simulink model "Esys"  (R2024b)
settings: Solver=ode15s  StartTime=0.0  StopTime=0.15  RelTol=1e-6  AbsTol=1e-6  EnableMultiTasking=on
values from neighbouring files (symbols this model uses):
  A = [-1 2; 0 -2]    [cds_matlab_intro_part3.m]    (also in Esys_Parameter.m = [A11,A12;A21,A22]; init_cds_simulink_intro_part1.m = [0 1; -1/T^2 -2*xi/T])
  B = [0;1]    [cds_matlab_intro_part3.m]    (also in init_cds_simulink_intro_part1.m = [0;V/T^2])
  D = 0    [cds_matlab_intro_part3.m]    (also in init_cds_simulink_intro_part1.m)
  te = 0.01    [Esys_Parameter.m]
  ts = 0.03    [Esys_Parameter.m]
  UC1R =     [Esys_Parameter.m]
  UC2R =     [Esys_Parameter.m]
  Ue = 1    [Esys_Parameter.m]
  UeR = 5    [Esys_Parameter.m]
  Us = 4    [Esys_Parameter.m]
  Usinus = 1    [Esys_Parameter.m]
  UsR = 5    [Esys_Parameter.m]
  we = 1e2    (= 100)    [Esys_Parameter.m]

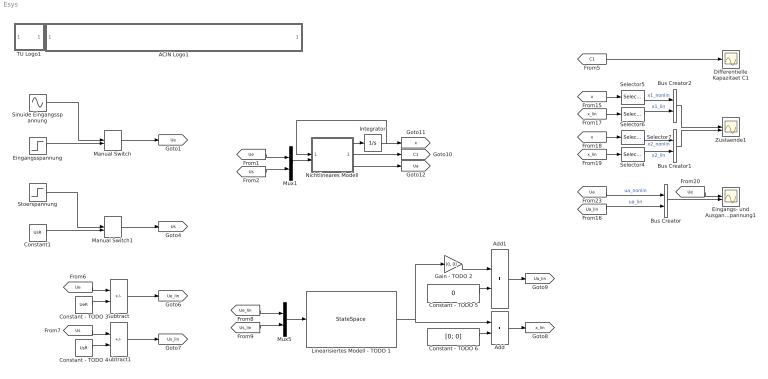
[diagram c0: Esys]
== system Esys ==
  ACIN Logo1 : Subsystem
      mask init:
      | s = get_param(gcb,'UserData');
  Add : Sum
  Add1 : Sum
  Bus Creator : BusCreator  Inputs=2
  Bus Creator1 : BusCreator  Inputs=2
  Bus Creator2 : BusCreator  Inputs=2
  Constant - TODO 3 : Constant  Value=UeR
  Constant - TODO 4 : Constant  Value=UsR
  Constant - TODO 5 : Constant  Value=0
  Constant - TODO 6 : Constant  Value=[0; 0]
  Constant1 : Constant  Value=UsR
  Differentielle Kapazitaet C1 : Scope
  Eingangs- und Ausgangsspannung1 : Scope  NumInputPorts=2
  Eingangsspannung : Step  Time=te  Before=UeR  After=Ue  SampleTime=0
  Gain - TODO 2 : Gain  Gain=[0, 0]  Multiplication=Matrix(K*u)
  Integrator : Integrator  InitialCondition=[UC1R; UC2R]
  Linearisiertes Modell - TODO 1 : StateSpace  A=A  B=B  C=eye(2)  D=[D;D]  InitialCondition=[0;0]
  Manual Switch : ManualSwitch
  Manual Switch1 : ManualSwitch  CurrentSetting=0
  Mux1 : Mux  Inputs=2
  Mux5 : Mux  Inputs=2
  Nichtlineares Modell : MATLAB Function  TreatAsAtomicUnit=on
  Selector4 : Selector  InputPortWidth=2  IndexOptions=Index vector (dialog)  Indices=2  OutputSizes=1
  Selector5 : Selector  InputPortWidth=2  IndexOptions=Index vector (dialog)  Indices=1  OutputSizes=1
  Selector6 : Selector  InputPortWidth=2  IndexOptions=Index vector (dialog)  Indices=1  OutputSizes=1
  Selector7 : Selector  InputPortWidth=2  IndexOptions=Index vector (dialog)  Indices=2  OutputSizes=1
  Sinuide Eingangsspannung : Sin  Amplitude=Usinus  Bias=UeR  Frequency=we  SampleTime=0
  Stoerspannung : Step  Time=ts  Before=UsR  After=Us  SampleTime=0
  Subtract : Sum  Inputs=+-
  Subtract1 : Sum  Inputs=+-
  TU Logo1 : Subsystem
      mask init:
      | s = get_param(gcb,'UserData');
  Zustaende1 : Scope  NumInputPorts=2
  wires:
  Eingangsspannung/1 -> Manual Switch/2
  Sinuide Eingangsspannung/1 -> Manual Switch/1
  Manual Switch/1 -> [Ue]
  [C1] -> Differentielle Kapazitaet C1/1
  Subtract/1 -> [Ue_lin]
  Constant - TODO 3/1 -> Subtract/2
  [Ue] -> Subtract/1
  Subtract1/1 -> [Us_lin]
  Constant - TODO 4/1 -> Subtract1/2
  [Us] -> Subtract1/1
  Linearisiertes Modell - TODO 1/1 -> Gain - TODO 2/1, Add/1
  Mux5/1 -> Linearisiertes Modell - TODO 1/1
  [Ue_lin] -> Mux5/1
  [Us_lin] -> Mux5/2
  Add/1 -> [x_lin]
  Constant - TODO 6/1 -> Add/2
  Gain - TODO 2/1 -> Add1/1
  Constant - TODO 5/1 -> Add1/2
  Add1/1 -> [Ua_lin]
  Manual Switch1/1 -> [Us]
  Stoerspannung/1 -> Manual Switch1/1
  Constant1/1 -> Manual Switch1/2
  Selector7/1 -> Bus Creator1/1  "x2_nonlin"
  Bus Creator/1 -> Eingangs- und Ausgangsspannung1/2
  Bus Creator1/1 -> Zustaende1/2
  Bus Creator2/1 -> Zustaende1/1
  [x_lin] -> Selector4/1
  [x] -> Selector7/1
  Selector6/1 -> Bus Creator2/2  "x1_lin"
  Selector5/1 -> Bus Creator2/1  "x1_nonlin"
  Selector4/1 -> Bus Creator1/2  "x2_lin"
  [Ua_lin] -> Bus Creator/2  "ua_lin"
  [x] -> Selector5/1
  [x_lin] -> Selector6/1
  [Ua] -> Bus Creator/1  "ua_nonlin"
  [Ue] -> Eingangs- und Ausgangsspannung1/1
  [Us] -> Mux1/2
  Mux1/1 -> Nichtlineares Modell/2(u)
  [Ue] -> Mux1/1
  Nichtlineares Modell/1(xp) -> Integrator/1
  Integrator/1 -> Nichtlineares Modell/1(x), [x]
  Nichtlineares Modell/2(C1) -> [C1]
  Nichtlineares Modell/3(Ua) -> [Ua]

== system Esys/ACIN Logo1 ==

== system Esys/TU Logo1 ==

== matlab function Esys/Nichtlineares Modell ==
function [xp, C1, Ua] = fcn(x, u, p)

R1 = p.R1;
R2 = p.R2;
K = p.K;
C1_ref  = p.C1_ref;
C1_inf  = p.C1_inf;
UC1_ref = p.UC1_ref;
C2      = p.C2;

% Shortcut fuer den Eingang
Ue = u(1);
Us = u(2);

% Shortcut fuer die Zustaende
UC1 = x(1);
UC2 = x(2);

% TODO
Ua = ; % Ausgangsspannung

% TODO: Erste Ableitung von Q1 nach UC1
dQ1 = ; % Aktueller Wert der differentiellen Kapazitaet C1
C1 = dQ1; 
% TODO: Berechnen der Zeitableitungen der Zustaende
xp = zeros(2,1);
xp(1) = ;
xp(2) = ;
